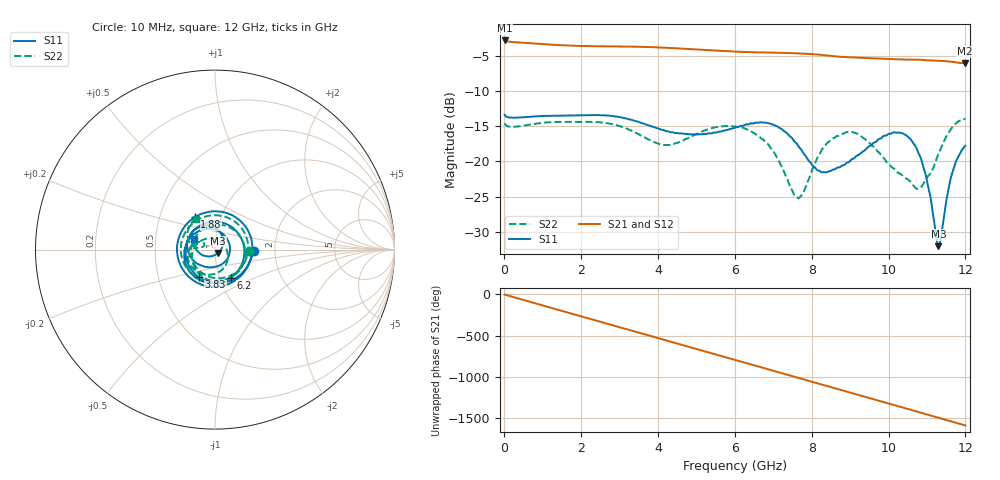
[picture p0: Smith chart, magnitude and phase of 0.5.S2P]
!Agilent Technologies,E5071C,MY46316741,A.11.02
!Date: Fri Apr 15 15:48:29 2022
!Data & Calibration Information:
!Freq	S11:SOLT2(ON)	S21:SOLT2(ON)	S12:SOLT2(ON)	S22:SOLT2(ON)
!PortZ  Port1:50+j0  Port2:50+j0
!Above PortZ is port z conversion or system Z0 setting when saving the data.
!When reading, reference impedance value at option line is always used.
# Hz S dB R 50
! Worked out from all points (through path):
!   1200 points, 10 MHz to 12 GHz, reference 50 ohm
!   highest |S21| = -2.77 dB at 10 MHz (marker M1); lowest = -6.0 dB at 11.99 GHz (marker M2)
!   group delay of S21, straight-line fit = 367 ps
!   lowest |S11| = -32.1 dB at 11.3 GHz (marker M3), VSWR 1.05, Z = 51.7 - j1.9 ohm
!   |S11| at or under -10 dB: start of sweep to end of sweep
!   |S22| runs from -25.2 to -13.9 dB; largest |S21 - S12| = 0.0043
!   S11 on the Smith chart (normalised r, x): 10 MHz: 1.55, -0.03; 1.88 GHz: 0.75, +0.28; 3.83 GHz: 0.80, -0.25; 6.2 GHz: 1.13, -0.36; 12 GHz: 0.79, +0.09
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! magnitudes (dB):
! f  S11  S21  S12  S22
! 10 MHz  -13.3  -2.8  -2.8  -14.5
! 1.88 GHz  -13.4  -3.5  -3.5  -14.4
! 2.01 GHz  -13.4  -3.6  -3.6  -14.4
! 3.83 GHz  -15.0  -3.7  -3.7  -17.1
! 4.01 GHz  -15.3  -3.8  -3.8  -17.5
! 4.96 GHz  -16.2  -4.0  -4.0  -16.2
! 6.01 GHz  -15.2  -4.4  -4.4  -15.0
! 6.2 GHz  -14.9  -4.4  -4.4  -15.2
! 6.92 GHz  -14.6  -4.5  -4.5  -18.0
! 7.61 GHz  -17.4  -4.6  -4.6  -25.1
! 7.76 GHz  -18.6  -4.6  -4.6  -24.6
! 8.01 GHz  -20.5  -4.7  -4.7  -21.2
! 8.4 GHz  -21.5  -4.9  -4.9  -17.4
! 8.95 GHz  -20.1  -5.1  -5.2  -15.8
! 10.01 GHz  -16.1  -5.4  -5.4  -20.4
! 10.43 GHz  -16.2  -5.5  -5.5  -22.3
! 10.77 GHz  -18.7  -5.5  -5.5  -23.9
! 11.01 GHz  -23.1  -5.6  -5.6  -22.2
! 11.3 GHz  -32.1  -5.6  -5.7  -18.9
! 11.65 GHz  -21.8  -5.8  -5.8  -15.2
! 11.99 GHz  -17.8  -6.0  -6.0  -13.9
! 12 GHz  -17.8  -6.0  -6.0  -13.9
